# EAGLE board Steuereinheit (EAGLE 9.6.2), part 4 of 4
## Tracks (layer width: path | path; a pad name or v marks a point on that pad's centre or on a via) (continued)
SE_WRITE_N  (via drill 0.35) (continued)
  Bottom 0.152: v123.85,59.79 v123.85,56.95 | v100.02,71.17 99.67,70.81 v99.67,68.68 | v81.18,68.5 v81.18,74.55 v81.18,78.1 | v66.95,82.73 v66.95,87.53 v66.95,92.69 v66.95,97.84 v66.95,102.82 66.95,108.33 v67.31,108.69
SE_WRITE_P  (via drill 0.35)
  Top 0.152: v114.07,57.48 114.25,57.3 114.25,55.35 PC_AN4.6 | 53.26,105.66 53.8,105.13 53.8,103.53 52.73,102.46 52.73,100.69 SE_BF3.1 52.55,100.69 v51.49,100.69 | 53.26,105.66 52.73,105.66 SE_BF2.1 53.26,105.66 | 53.26,110.64 52.73,110.64 SE_BF1.1 53.26,110.64 | 53.26,110.64 54.15,109.75 54.15,106.55 53.26,105.66 | 53.44,115.62 53.8,115.26 53.8,111.18 53.26,110.64 | 53.44,115.62 53.26,115.8 52.73,115.8 SE_BF0.1 | v51.49,81.84 52.55,80.77 52.55,80.42 SE_BF7.1 | v51.49,85.22 52.38,85.22 52.55,85.4 SE_BF6.1 52.73,85.57 53.8,86.64 53.8,89.84 53.26,90.37 52.73,90.37 SE_BF5.1 | v51.49,95.53 52.55,95.53 SE_BF4.1 | v14.86,64.06 13.44,64.06 11.48,62.1 11.48,61.57 SE_JK2.15 | v47.22,38.81 46.51,38.1 46.51,36.14 M_OR1.8 | v84.56,115.44 76.02,115.44 72.82,118.64 56.46,118.64 53.44,115.62
  Route2 0.152: v14.86,64.06 30.15,64.06 40.11,74.02 43.66,74.02 v51.49,81.84
  Route15 0.152: v114.07,57.48 113.54,57.48 112.29,58.73 109.8,58.73 100.38,68.15 100.38,69.75 95.4,74.73 95.4,80.42 93.98,81.84 93.98,88.95 86.51,96.42 M48Z08.22
  Bottom 0.152: v47.22,38.81 46.86,39.17 46.86,58.9 47.22,59.26 47.22,63.35 46.86,63.7 46.86,64.59 47.22,64.95 47.22,75.08 46.86,75.44 46.86,77.22 v51.49,81.84 v51.49,85.22 v51.49,95.53 v51.49,100.69 | v84.56,115.44 84.56,98.37 86.33,96.6 M48Z08.22
SP_N0  (via drill 0.35)
  Top 0.152: v74.78,114.38 74.42,114.02 70.69,114.02 68.02,116.69 65.53,116.69 64.82,115.98 63.58,115.98 SP_BF0.4 | v74.95,40.77 73.71,39.52 73.71,38.63 BR_NO2.11 | v80.29,27.25 81.18,26.37 81.18,24.77 BR_AN3.13 | v57,76.15 54.33,76.15 52.55,74.37 52.55,71.88 53.26,71.17 53.26,66.9 BR_OR2.1 | v84.56,42.19 85.27,42.19 86.33,43.26 86.33,43.79 BR_JK1.6 | v100.56,53.57 98.96,53.57 97.89,54.63 97.89,55.35 BR_NO1.5 | v127.05,46.81 127.94,46.81 128.83,45.92 128.83,45.21 BR_JK3.6
  Route2 0.152: v74.95,40.77 76.38,42.19 v84.56,42.19 88.82,46.46 95.05,46.46 97.71,49.12 98.25,49.12 101.27,52.15 101.27,52.86 v100.56,53.57
  Route15 0.152: v57,76.15 60.38,76.15 61.44,75.08 74.6,75.08 v74.78,74.91 | v127.05,46.81 126.34,46.81 118.16,54.99 111.23,54.99 109.27,53.04 102.16,53.04 100.91,51.79 100.2,51.79 99.85,52.15 99.85,52.86 v100.56,53.57
  Bottom 0.152: v74.78,114.38 v74.78,74.91 74.78,56.77 74.42,56.41 74.42,48.41 74.95,47.88 v74.95,40.77 75.84,39.88 75.84,31.7 v80.29,27.25
SP_N1  (via drill 0.35)
  Top 0.152: v129.36,35.43 129.01,35.08 129.01,33.83 BR_JK7.6 | v129.36,46.81 129.36,49.84 130.07,50.55 130.07,51.26 BR_JK3.10 | 63.04,116.87 63.22,117.04 73.89,117.04 76.91,114.02 88.11,114.02 v92.02,110.11 | 63.04,116.87 62.51,116.33 62.51,115.44 62.86,115.09 63.75,115.09 64.47,114.38 64.47,113.49 63.58,112.6 63.58,110.82 SP_BF1.4 | v91.67,61.39 91.67,62.28 92.38,62.99 94.34,62.99 95.22,62.1 95.22,61.57 BR_NO1.14 | v49.17,89.66 49.71,89.13 49.71,68.5 52.91,65.3 53.8,65.3 54.51,66.02 54.51,66.73 BR_OR2.2 | 63.04,116.87 v63.04,117.93 | v90.25,27.96 89,27.96 86.51,25.48 86.51,24.77 BR_AN3.9 | BR_NO2.9 78.87,38.63 v79.05,38.81
  Route2 0.152: v49.17,89.66 49.17,90.19 59.84,100.86 59.84,114.73 v63.04,117.93
  Route15 0.152: v79.05,38.81 89.89,38.81 v90.25,38.46 | v129.36,35.43 129.36,36.32 130.96,37.92 130.96,38.63 130.61,38.99 129.36,38.99 115.85,25.48 92.73,25.48 v90.25,27.96
  Bottom 0.152: v129.36,46.81 v129.36,35.43 | 92.02,72.06 92.02,64.24 91.67,63.88 v91.67,61.39 | 92.02,72.06 v92.02,110.11 | v90.25,27.96 v90.25,38.46 90.25,40.41 89,41.66 89,71.7 89.36,72.06 92.02,72.06
SP_N2  (via drill 0.35)
  Top 0.152: v130.25,38.28 130.25,39.88 BR_JK7.10 | v141.28,46.81 141.81,46.81 142.88,45.75 BR_JK4.6 | v91.14,18.9 89.36,17.12 87.05,17.12 86.51,17.65 86.51,18.36 BR_AN3.6 | v91.49,54.28 91.49,56.06 92.02,56.59 | 92.02,56.59 93.09,57.66 93.8,57.66 96.29,60.15 98.42,60.15 98.96,60.68 98.96,61.39 BR_NO1.11 | v62.33,105.13 62.86,105.66 63.4,105.66 SP_BF2.4 | v59.31,68.5 58.42,67.62 BR_OR2.5 | v20.19,47.88 19.3,46.99 16.1,46.99 15.04,45.92 15.04,45.21 15.21,45.03 15.21,43.97 BR_NO3.5 | 92.02,56.59 91.67,56.95 v91.49,56.95
  Route2 0.152: v130.25,38.28 132.74,38.28 v141.28,46.81 | v62.33,105.13 62.33,104.78 68.2,98.91 68.2,77.39 v59.31,68.5 58.6,67.79 56.82,67.79 51.66,62.64 40.82,62.64 37.26,59.08 32.99,59.08 23.57,49.66 21.97,49.66 v20.19,47.88
  Route15 0.152: v130.25,38.28 130.25,37.74 113.54,21.03 93.27,21.03 v91.14,18.9 | v91.49,56.95 86.87,56.95 86.51,56.59 71.93,56.59 60.02,68.5 v59.31,68.5
  Bottom 0.152: v91.14,18.9 91.14,53.92 v91.49,54.28
SP_N3  (via drill 0.35)
  Top 0.152: BR_JK8.6 142.88,34.37 v144.12,35.61 | v144.12,48.06 144.12,51.26 BR_JK4.10 | v62.51,99.44 62.51,99.62 63.4,100.51 SP_BF3.4 | v59.66,65.13 59.66,66.73 BR_OR2.6 | v12.55,45.75 12.55,43.97 BR_NO3.3 | v81.71,20.14 81.36,19.79 81.36,18.54 BR_AN3.2 | v101.62,63.35 101.62,61.57 BR_NO1.9
  Route15 0.152: v62.51,99.44 60.2,97.13 59.49,97.13 53.98,91.62 53.98,76.86 | 53.98,68.68 53.98,76.86 | 53.98,68.68 57.53,65.13 v59.66,65.13 | v12.55,45.75 19.66,52.86 20.37,52.86 27.3,59.79 27.3,60.15 30.15,62.99 34.59,62.99 39.39,67.79 53.09,67.79 53.98,68.68 | v81.71,20.14 72.82,29.03 71.75,29.03 62.86,37.92 62.86,38.28 v60.73,40.41 | v101.62,63.35 101.09,63.35 95.58,68.86 89.36,68.86 84.56,73.66 79.22,73.66 76.02,76.86 53.98,76.86 | v144.12,35.61 143.23,35.61 141.63,37.21 135.94,37.21 128.65,44.5 104.65,44.5 v102.34,46.81
  Bottom 0.152: v144.12,48.06 v144.12,35.61 | v60.73,40.41 60.73,51.26 61.09,51.61 61.09,63.7 v59.66,65.13 | v102.34,46.81 101.27,47.88 101.27,62.99 v101.62,63.35
SP_N4  (via drill 0.35)
  Top 0.152: v62.15,94.82 62.86,95.53 63.4,95.53 SP_BF4.4 | v46.33,65.13 46.33,62.1 BR_AA4.9 | v14.33,45.57 12.72,47.17 12.72,50.01 BR_NO3.14 | v75.49,30.81 70.87,30.81 69.98,31.7 69.98,32.41 BR_NO2.3 | v81,34.9 81.36,34.9 81.89,35.43 87.94,35.43 89.71,33.66 89.71,31.34 88.82,30.45 | 88.82,30.45 87.58,30.45 86.51,31.52 86.51,32.41 BR_JK5.6 | 93.98,25.3 BR_AN4.13 93.98,24.77 | 88.82,30.45 93.98,25.3 | v103.05,44.14 103.4,44.5 103.4,55.52 102.16,56.77 101.09,56.77 100.38,56.06 100.38,55.35 BR_NO1.7 | v103.05,26.54 95.22,26.54 93.98,25.3 | v121.54,32.23 124.56,32.23 126.16,30.63 138.43,30.63 139.32,31.52 145.01,31.52 146.08,32.59 146.08,41.12 145.9,41.3 144.83,41.3 144.3,40.77 144.3,40.06 BR_JK8.10
  Route2 0.152: v62.15,94.82 62.15,93.22 61.27,92.33 61.27,88.24 60.02,87 60.02,80.24 46.33,66.55 v46.33,65.13 | v81,34.9 76.91,30.81 v75.49,30.81 75.49,26.19 74.78,25.48 70.87,25.48 58.6,37.74 45.8,37.74 43.48,40.06 32.46,40.06 29.97,42.55 17.7,42.55 14.68,45.57 v14.33,45.57
  Route15 0.152: v14.33,45.57 14.33,46.63 15.93,48.23 15.93,48.59 19.84,52.5 21.79,52.5 29.44,60.15 32.28,60.15 36.55,64.41 45.62,64.41 v46.33,65.13 | v121.54,32.23 115.14,25.83 103.76,25.83 v103.05,26.54
  Bottom 0.152: v103.05,26.54 v103.05,44.14
SP_N5  (via drill 0.35)
  Top 0.152: v88.11,40.23 87.76,39.88 87.76,38.63 BR_JK5.10 | v89,22.28 91.85,22.28 92.73,21.39 97.54,21.39 98.96,22.81 98.96,24.59 BR_AN4.9 | BR_AA2.10 58.42,51.44 v58.78,51.79 | 58.42,56.95 56.82,56.95 55.93,56.06 55.93,55.35 BR_AA3.3 | 58.42,56.95 BR_AA3.10 | 58.42,56.95 v58.78,56.95 | v56.64,89.31 58.06,90.73 61.44,90.73 61.62,90.55 63.4,90.55 SP_BF5.4 | v42.06,74.73 42.06,72.95 BR_NO4.14 41.88,72.77 41.88,72.24 41.17,71.53 39.39,71.53 37.97,70.1 37.97,55.7 34.42,52.15 23.39,52.15 21.97,53.57 v20.02,53.57 | v20.02,51.44 17.17,51.44 16.64,50.9 16.64,50.19 BR_NO3.11 | v41.35,56.95 41.88,56.41 41.88,55.35 BR_AA4.3
  Route2 0.152: v42.06,74.73 v56.64,89.31 | v58.78,56.95 57.53,56.95 56.82,57.66 42.06,57.66 v41.35,56.95
  Route15 0.152: v88.11,40.23 83.13,40.23 76.73,46.63 63.93,46.63 v58.78,51.79
  Bottom 0.152: v88.11,40.23 88.82,39.52 88.82,23.52 89,23.34 v89,22.28 | v58.78,56.95 v58.78,51.79 | v20.02,53.57 v20.02,51.44 | v41.35,56.95 41.17,57.12 41.17,62.99 41.88,63.7 41.88,74.55 v42.06,74.73
SP_N6  (via drill 0.35)
  Top 0.152: v21.26,47.88 19.13,50.01 BR_NO3.9 | v33.71,47.88 37.44,47.88 37.8,47.52 41.71,47.52 43.13,48.95 43.13,50.01 BR_AA1.11 43.31,50.19 43.31,50.9 44.2,51.79 v47.57,51.79 | v99.14,20.14 99.14,18.54 BR_AN4.6 | v99.14,29.21 99.14,32.41 BR_JK6.6 | v58.78,85.93 61.09,85.93 61.44,85.57 63.4,85.57 SP_BF6.4 | v47.57,75.79 47.57,75.44 45.8,73.66 45.8,72.95 BR_NO4.11 | v47.57,64.06 47.75,63.88 47.75,59.79 46.86,58.9 45.09,58.9 43.31,57.12 43.31,55.35 BR_AA4.4 | v47.93,45.39 56.29,45.39 57,44.68 57,43.97 BR_AA2.4 | v51.31,59.44 55.75,59.44 57,60.68 57,61.39 BR_AA3.11
  Route2 0.152: v33.71,47.88 v21.26,47.88 | v58.78,85.93 57.71,85.93 v47.57,75.79
  Route15 0.152: v99.14,29.21 98.42,29.92 83.84,29.92 77.8,35.97 75.49,35.97 69.98,41.48 68.38,41.48 65,44.86 48.46,44.86 v47.93,45.39
  Bottom 0.152: v99.14,29.21 v99.14,20.14 | v47.57,75.79 v47.57,64.06 47.57,59.44 | v47.93,45.39 47.57,45.75 v47.57,51.79 47.57,59.44 | 47.57,59.44 v51.31,59.44
SP_N7  (via drill 0.35)
  Top 0.152: v93.98,20.32 BR_AN4.2 | v98.96,37.03 99.31,37.03 100.2,37.92 100.2,38.63 BR_JK6.10 | v56.64,82.55 60.2,82.55 62.33,80.42 63.4,80.42 SP_BF7.4 | v48.64,74.55 48.64,73.3 BR_NO4.9 | v22.86,41.12 21.44,42.55 18.59,42.55 17.88,43.26 17.88,43.79 BR_NO3.7 | v47.93,42.55 45.26,42.55 44.55,43.26 44.55,43.79 BR_AA1.5 | v47.93,40.59 48.11,40.41 53.62,40.41 55.04,41.83 57,41.83 58.42,43.26 BR_AA2.5 58.42,44.5 59.49,45.57 v60.02,45.57 | BR_AA4.5 44.55,55.35 44.55,54.63 45.26,53.92 48.11,53.92 v48.28,54.1 48.28,56.77 49,57.48 49,64.24 48.64,64.59 v48.64,65.13 | BR_AA3.5 58.42,53.92 v60.38,51.97
  Route2 0.152: v93.98,20.32 93.98,27.43 95.05,28.5 95.05,29.92 94.16,30.81 94.16,33.3 93.09,34.37 93.09,35.08 94.34,36.32 98.25,36.32 v98.96,37.03 | v48.64,74.55 v56.64,82.55
  Route15 0.152: v22.86,41.12 28.73,41.12 29.26,41.66 30.86,41.66 31.04,41.48 39.57,41.48 40.64,42.55 v47.93,42.55 | v98.96,37.03 96.83,39.17 82.07,39.17 77.09,44.14 66.24,44.14 65.18,45.21 60.38,45.21 v60.02,45.57
  Bottom 0.152: v47.93,40.59 v47.93,42.55 47.93,44.14 48.64,44.86 48.64,45.75 48.28,46.1 v48.28,54.1 | v60.38,51.97 60.38,45.92 v60.02,45.57 | v48.64,65.13 v48.64,74.55
USB_4
  Top 0.152: R12.1 12.37,13.92 12.37,8.76 X2.1

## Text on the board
Top: created by Moritz Prünster 2023/24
